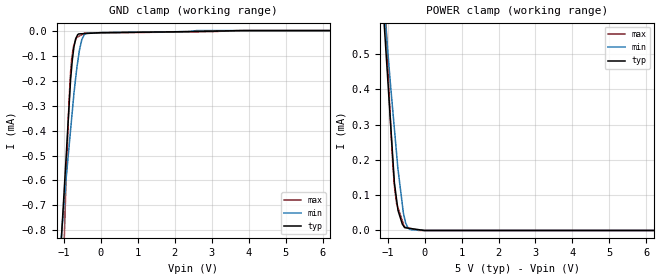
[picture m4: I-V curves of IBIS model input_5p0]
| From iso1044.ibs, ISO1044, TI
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|   input_5p0 Model
[Model]   input_5p0
Model_type   Input
Vinl = 1.5
Vinh = 3.5
|   typ   min   max
C_comp   0.001pF   0.0008pF   0.0178pF
|  Where Nom  PVT is Nominal Process, 5V,   27C
|   Fast PVT is Strong Process,  5.5V,  -40C
|   Slow PVT is Weak Process,   4.5V,   150C
[Model spec]
|subparameter
Vinl   1.5   1.35   1.65
Vinh   3.5   3.15   3.85
[Voltage Range]   5   4.5   5.5
|Junction Temperature
[Temperature Range]   27   150   -40
[Power Clamp Reference]   5   4.5   5.5
[GND Clamp Reference]   0   0   0
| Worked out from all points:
|   GND clamp passes 1 mA (typ) near -1.13 V on its own axis
[GND Clamp]
|   Voltage   I(typ)   I(min)   I(max)
-5V       -12.41mA   -8.478mA   -24.5mA
-1.131V   -992.2uA   -935.6uA   -1.543mA
-1.028V   -729.6uA   -747.9uA   -1.012mA
-944.9mV  -517.6uA   -601.5uA   -615.4uA
-880.7mV  -353.5uA   -496.1uA   -349.4uA
-818.5mV  -194.4uA   -396uA     -163.9uA
-790.6mV  -148uA     -351.2uA   -113.2uA
-727.8mV  -64.6uA    -250.3uA   -57.62uA
-602.7mV  -13.49uA   -101.1uA   -23.73uA
-515.5mV  -12.73uA   -35.9uA    -16.43uA
-387mV    -11.62uA   -10.54uA   -10.06uA
10V       0A         0A         0A
[POWER Clamp]
|   Voltage   I(typ)   I(min)   I(max)
-5V       97.6mA     38.05mA    157.6mA
-1.128V   640.5uA    684.1uA    812.9uA
-1.035V   488.7uA    558.3uA    562.9uA
-941mV    335.9uA    436.1uA    342.9uA
-863.2mV  208.8uA    342uA      191.5uA
-811mV    129.7uA    280uA      119.2uA
-720.2mV  56.8uA     173.3uA    64.07uA
-576mV    13.8uA     50.27uA    18.7uA
-537.2mV  7.914uA    32.01uA    9.786uA
-387mV    5.701uA    2.389uA    5.885uA
-104.8uV  1.273nA    0A         162.1fA
10V       0A         0A         0A
